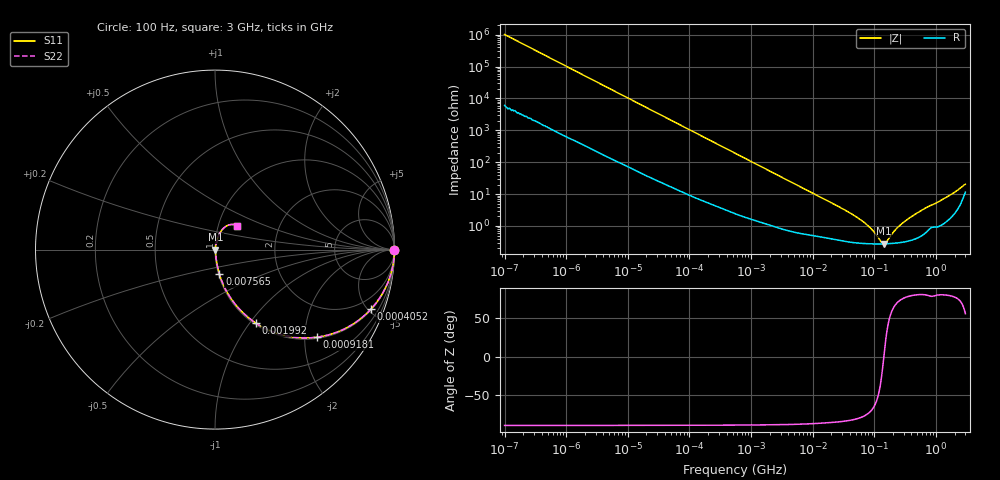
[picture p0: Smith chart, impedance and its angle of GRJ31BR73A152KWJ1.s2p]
!Murata Part Number: GRJ31BR73A152KWJ1
!These Parameters are Measured in Series Mode Connection
!Data Generated on Jun 19, 2026
!  o--ll--o
!Port1  Port2
!  o------o
!Operation Temp=25[degC], DC Bias Voltage=0[V]
!Freq. Start=100[Hz] Stop=3[GHz] 401[Steps]
# Hz S RI R 50
!Freq.(Hz) S11(Real) S11(Imag) S21(Real) S21(Imag) S12(Real) S12(Imag) S22(Real) S22(Imag)
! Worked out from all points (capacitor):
!   401 points, 100 Hz to 3 GHz, reference 50 ohm
!   read as one part in series: C = 1.57 nF near 109 Hz
!   lowest |Z| = 276 mohm at 141.2 MHz (marker M1)
!   series resonance near 142.6 MHz, so ESL is about 790 pH
!   S11 on the Smith chart (normalised r, x): 100 Hz: open; 405.2 kHz: 1.06, -5.19; 918.1 kHz: 1.03, -2.30; 1.992 MHz: 1.02, -1.07; 7.565 MHz: 1.01, -0.28; 3 GHz: 1.23, +0.34
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100  1 -9.87e-05  6e-07 9.87e-05  6e-07 9.87e-05  1 -9.87e-05
1788  1 -0.00175  1.43e-05 0.00175  1.43e-05 0.00175  1 -0.00175
31977  0.9988 -0.0308  0.00119 0.0308  0.00119 0.0308  0.9988 -0.0308
132342  0.9831 -0.1244  0.0169 0.1244  0.0169 0.1244  0.9831 -0.1244
405239  0.8678 -0.3329  0.1322 0.3329  0.1322 0.3329  0.8678 -0.3329
547723  0.7843 -0.405  0.2157 0.405  0.2157 0.405  0.7843 -0.405
918067  0.5691 -0.4878  0.4309 0.4878  0.4309 0.4878  0.5691 -0.4878
1992254  0.2266 -0.4088  0.7734 0.4088  0.7734 0.4088  0.2266 -0.4088
3486191  0.0918 -0.2765  0.9082 0.2765  0.9082 0.2765  0.0918 -0.2765
7565221  0.0249 -0.1378  0.9751 0.1378  0.9751 0.1378  0.0249 -0.1378
9794414  0.0168 -0.1076  0.9832 0.1076  0.9832 0.1076  0.0168 -0.1076
2.999103e7  0.00462 -0.035  0.9954 0.035  0.9954 0.035  0.00462 -0.035
5.719833e7  0.00314 -0.0163  0.9969 0.0163  0.9969 0.0163  0.00314 -0.0163
8.425944e7  0.00283 -0.0086  0.9972 0.0086  0.9972 0.0086  0.00283 -0.0086
1.295826e8  0.00274 -0.00149  0.9973 0.00149  0.9973 0.00149  0.00274 -0.00149
1.412317e8  0.00275 -0.000145  0.9973 0.000145  0.9973 0.000145  0.00275 -0.000145
1.539281e8  0.00276 0.0012  0.9972 -0.0012  0.9972 -0.0012  0.00276 0.0012
1.751444e8  0.0028 0.00325  0.9972 -0.00325  0.9972 -0.00325  0.0028 0.00325
2.471375e8  0.00304 0.00906  0.997 -0.00906  0.997 -0.00906  0.00304 0.00906
3.800727e8  0.00379 0.018  0.9962 -0.018  0.9962 -0.018  0.00379 0.018
1.71441e9  0.0254 0.089  0.9746 -0.089  0.9746 -0.089  0.0254 0.089
3e9  0.1236 0.1339  0.8764 -0.1339  0.8764 -0.1339  0.1236 0.1339
